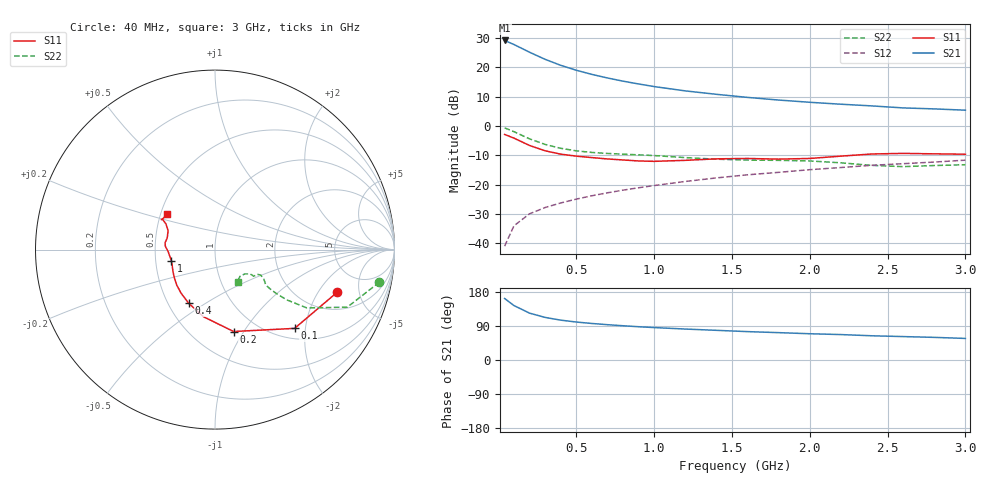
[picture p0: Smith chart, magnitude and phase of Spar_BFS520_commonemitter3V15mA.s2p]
! Filename:  BFS520D.S2P  Version:  4.0
! NXP part #: BFS520  Date: Jun 1994
! Bias condition: Vce=3V, Ic=15mA
#  MHz  S  MA  R  50
! Freq  S11  S21  S12  S22  !GUM [dB]
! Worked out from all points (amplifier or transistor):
!   21 points, 40 MHz to 3 GHz, reference 50 ohm
!   highest |S21| = 29.2 dB at 40 MHz (marker M1)
!   |S21| within 3 dB of that: start of sweep to 161.7 MHz
!   unconditionally stable (mu >= 1): 712.6 MHz to end of sweep
!   at 300 MHz: K = 0.74, MSG = 25.3 dB, |S12| = -27.7 dB
!   at 1 GHz: K = 1.07, MAG = 15.2 dB, |S12| = -20.3 dB
!   at 3 GHz: K = 1.05, MAG = 7.2 dB, |S12| = -11.6 dB
!   lowest NFmin = 1.30 dB at 500 MHz
!   S11 on the Smith chart (normalised r, x): 40 MHz: 3.05, -3.01; 100 MHz: 1.22, -1.75; 200 MHz: 0.77, -0.90; 400 MHz: 0.63, -0.43; 1 GHz: 0.60, -0.08; 3 GHz: 0.54, +0.24
40  0.722 -19.1  28.82 162.3  0.009 80.4  0.934 -11.2
100  0.624 -44.7  24.59 143.7  0.02 70.1  0.804 -23.5
200  0.468 -77.2  18.17 123.7  0.032 63.0  0.607 -32.4
300  0.38 -99.5  13.75 112.4  0.041 62.8  0.488 -35.0
400  0.333 -116.1  10.88 105.2  0.049 64.1  0.419 -35.6
500  0.308 -127.7  8.966 100.2  0.057 65.5  0.379 -35.5
600  0.291 -137.0  7.618 96.4  0.065 67.1  0.356 -35.1
700  0.276 -145.0  6.619 93.2  0.073 68.5  0.342 -34.5
800  0.265 -151.8  5.841 90.4  0.081 69.6  0.333 -33.3
900  0.255 -159.0  5.231 87.8  0.089 70.4  0.324 -32.0
1000  0.251 -165.8  4.723 85.6  0.097 70.9  0.315 -30.7
1200  0.261 -177.4  3.986 81.7  0.114 71.8  0.291 -29.1
1400  0.277 176.3  3.485 78.3  0.131 72.5  0.273 -30.3
1600  0.281 172.1  3.087 74.9  0.148 72.2  0.264 -33.7
1800  0.274 166.7  2.782 72.2  0.163 72.5  0.261 -34.7
2000  0.281 158.3  2.548 69.3  0.181 72.3  0.255 -34.4
2200  0.308 152.4  2.362 67.1  0.197 72.4  0.237 -34.8
2400  0.335 150.2  2.21 63.9  0.215 72.0  0.214 -39.3
2600  0.343 150.8  2.043 61.8  0.229 71.0  0.204 -47.0
2800  0.337 149.0  1.965 59.7  0.244 71.1  0.213 -52.4
3000  0.332 143.5  1.869 56.9  0.263 70.4  0.22 -54.2
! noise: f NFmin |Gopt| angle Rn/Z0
500  1.3  0.098  37  0.2
900  1.45  0.075  99  0.18
2000  2.05  0.265  -158  0.18
